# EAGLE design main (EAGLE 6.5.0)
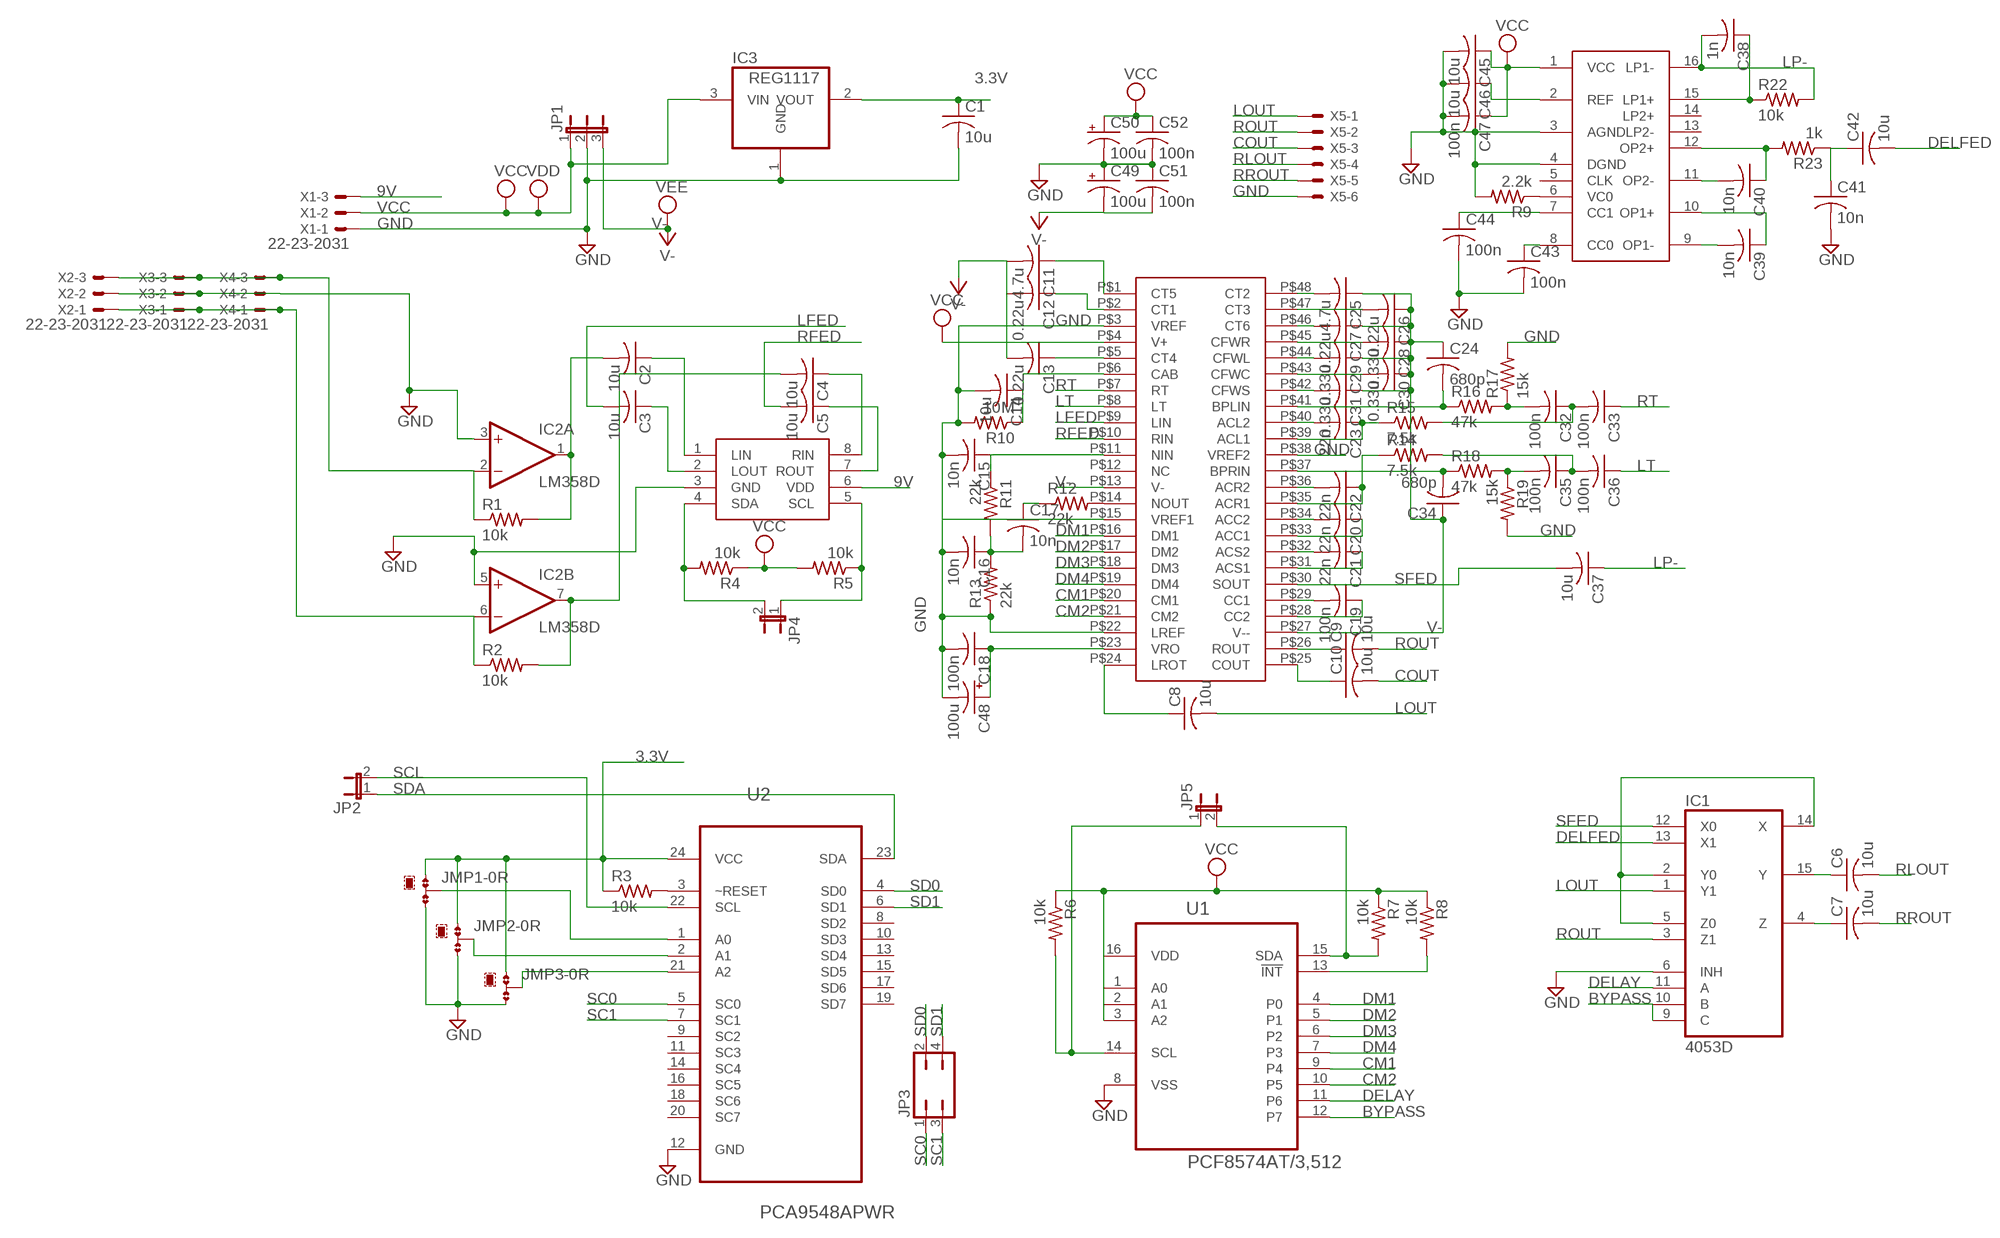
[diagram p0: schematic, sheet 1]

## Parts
C1  10u  C-USC1206  [C1206]
C2  10u  C-USC1206  [C1206]
C3  10u  C-USC1206  [C1206]
C4  10u  C-USC1206  [C1206]
C5  10u  C-USC1206  [C1206]
C6  10u  C-USC1206  [C1206]
C7  10u  C-USC1206  [C1206]
C8  10u  C-USC1206  [C1206]
C9  10u  C-USC1206  [C1206]
C10  10u  C-USC1206  [C1206]
C11  4.7u  C-USC1206  [C1206]
C12  0.22u  C-USC1206  [C1206]
C13  0.22u  C-USC1206  [C1206]
C14  10u  C-USC1206  [C1206]
C15  10n  C-USC1206  [C1206]
C16  10n  C-USC1206  [C1206]
C17  10n  C-USC1206  [C1206]
C18  100n  C-USC1206  [C1206]
C19  100n  C-USC1206  [C1206]
C20  22n  C-USC1206  [C1206]
C21  22n  C-USC1206  [C1206]
C22  22n  C-USC1206  [C1206]
C23  22n  C-USC1206  [C1206]
C24  680p  C-USC1206  [C1206]
C25  4.7u  C-USC1206  [C1206]
C26  0.22u  C-USC1206  [C1206]
C27  0.22u  C-USC1206  [C1206]
C28  0.33u  C-USC1206  [C1206]
C29  0.33u  C-USC1206  [C1206]
C30  0.33u  C-USC1206  [C1206]
C31  0.33u  C-USC1206  [C1206]
C32  100n  C-USC1206  [C1206]
C33  100n  C-USC1206  [C1206]
C34  680p  C-USC1206  [C1206]
C35  100n  C-USC1206  [C1206]
C36  100n  C-USC1206  [C1206]
C37  10u  C-USC1206  [C1206]
C38  1n  C-USC1206  [C1206]
C39  10n  C-USC1206  [C1206]
C40  10n  C-USC1206  [C1206]
C41  10n  C-USC1206  [C1206]
C42  10u  C-USC1206  [C1206]
C43  100n  C-USC1206  [C1206]
C44  100n  C-USC1206  [C1206]
C45  10u  C-USC1206  [C1206]
C46  10u  C-USC1206  [C1206]
C47  100n  C-USC1206  [C1206]
C48  100u  CPOL-USE2-5  [E2-5]
C49  100u  CPOL-USE2-5  [E2-5]
C50  100u  CPOL-USE2-5  [E2-5]
C51  100n  C-USC1206  [C1206]
C52  100n  C-USC1206  [C1206]
IC1  4053D  [SO16]
IC2  LM358D  [SO08]
IC3  REG1117  [SOT223]
JMP1  0R-JUMPB  [B0R-JMP]
JMP2  0R-JUMPB  [B0R-JMP]
JMP3  0R-JUMPB  [B0R-JMP]
JP1  JP2W  [JP2W]
JP2  JP1E  [JP1]
JP3  JP2Q  [JP2Q]
JP4  JP1E  [JP1]
JP5  JP1E  [JP1]
R1  10k  R-US_R1206  [R1206]
R2  10k  R-US_R1206  [R1206]
R3  10k  R-US_R1206  [R1206]
R4  10k  R-US_R1206  [R1206]
R5  10k  R-US_R1206  [R1206]
R6  10k  R-US_R1206  [R1206]
R7  10k  R-US_R1206  [R1206]
R8  10k  R-US_R1206  [R1206]
R9  2.2k  R-US_R1206  [R1206]
R10  10M  R-US_R1206  [R1206]
R11  22k  R-US_R1206  [R1206]
R12  22k  R-US_R1206  [R1206]
R13  22k  R-US_R1206  [R1206]
R14  7.5k  R-US_R1206  [R1206]
R15  7.5k  R-US_R1206  [R1206]
R16  47k  R-US_R1206  [R1206]
R17  15k  R-US_R1206  [R1206]
R18  47k  R-US_R1206  [R1206]
R19  15k  R-US_R1206  [R1206]
R22  10k  R-US_R1206  [R1206]
R23  1k  R-US_R1206  [R1206]
U1  PCF8574AT/3,512  [SOIC127P1032X265-16N]
U2  PCA9548APWR  [SOP65P640X120-24N]
U$1  SSM2126  [DIP48]
U$2  PT2257  [SO08]
U$3  PT2399  [DIL16]
X1  22-23-2031  [22-23-2031]
X2  22-23-2031  [22-23-2031]
X3  22-23-2031  [22-23-2031]
X4  22-23-2031  [22-23-2031]
X5  22-23-2061  [22-23-2061]

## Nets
3.3V: C1.1 IC3.2(VOUT) JMP1.1 JMP2.1 JMP3.1 R3.1 U2.24(VCC)
9V: U$2.6(VDD) X1.3
BYPASS: IC1.9(C) IC1.10(B) U1.12(P7)
CM1: U1.9(P4) U$1.P$20(CM1)
CM2: U1.10(P5) U$1.P$21(CM2)
COUT: C10.2 X5.3
DELAY: IC1.11(A) U1.11(P6)
DELFED: C42.2 IC1.13(X1)
DM1: U1.4(P0) U$1.P$16(DM1)
DM2: U1.5(P1) U$1.P$17(DM2)
DM3: U1.6(P2) U$1.P$18(DM3)
DM4: U1.7(P3) U$1.P$19(DM4)
GND: C1.2 C14.2 C15.2 C16.2 C18.2 C41.2 C43.2 C44.2 C45.2 C46.2 C47.2 C48.- C49.+ C50.- C51.1 C52.2 IC1.6(INH) IC2.3(A:+IN) IC2.5(B:+IN) IC3.1(GND) JMP1.3 JMP2.3 JMP3.3 JP1.2 R9.2 R10.2 R13.1 R17.2 R19.2 U1.8(VSS) U2.12(GND) U$1.P$3(VREF) U$1.P$15(VREF1) U$1.P$22(LREF) U$1.P$38(VREF2) U$2.3(GND) U$3.3(AGND) U$3.4(DGND) X1.1 X2.2 X3.2 X4.2 X5.6
LFED: C3.2 U$1.P$9(LIN)
LOUT: C8.2 IC1.1(Y1) X5.1
LP-: C37.1 C38.2 R22.2 U$3.16(LP1-)
LT: C36.1 U$1.P$8(LT)
N$1: R3.2 U2.3(~RESET)
N$2: C2.2 IC2.1(A:OUT) R1.2
N$3: IC2.2(A:-IN) R1.1 X2.3 X3.3 X4.3
N$4: IC2.6(B:-IN) R2.1 X2.1 X3.1 X4.1
N$5: C4.2 IC2.7(B:OUT) R2.2
N$6: C11.1 U$1.P$1(CT5)
N$7: R9.1 U$3.6(VC0)
N$8: C2.1 U$2.1(LIN)
N$9: C4.1 U$2.8(RIN)
N$10: C3.1 U$2.2(LOUT)
N$11: C5.1 U$2.7(ROUT)
N$12: JMP2.2 U2.2(A1)
N$13: JMP3.2 U2.21(A2)
N$14: JMP1.2 U2.1(A0)
N$15: IC1.2(Y0) IC1.5(Z0) IC1.14(X)
N$16: C6.1 IC1.15(Y)
N$17: C7.1 IC1.4(Z)
N$18: R8.2 U1.13(!INT)
N$19: C8.1 U$1.P$24(LROT)
N$20: C12.1 U$1.P$2(CT1)
N$21: C9.1 U$1.P$26(ROUT)
N$22: C10.1 U$1.P$25(COUT)
N$23: C13.1 U$1.P$5(CT4)
N$24: C14.1 R10.1 U$1.P$6(CAB)
N$25: R12.2 U$1.P$14(NOUT)
N$26: C15.1 R11.1 U$1.P$11(NIN)
N$27: C16.1 C17.2 R11.2 R13.2
N$28: C17.1 R12.1
N$29: C19.2 U$1.P$29(CC1)
N$30: C18.1 C48.+ U$1.P$23(VRO)
N$31: C19.1 U$1.P$28(CC2)
N$32: C21.1 U$1.P$31(ACS1)
N$33: C21.2 U$1.P$32(ACS2)
N$34: C20.1 U$1.P$33(ACC1)
N$35: C20.2 U$1.P$34(ACC2)
N$36: C22.1 R14.1 U$1.P$35(ACR1)
N$37: C22.2 U$1.P$36(ACR2)
N$38: C23.2 U$1.P$40(ACL2)
N$39: C23.1 R15.1 U$1.P$39(ACL1)
N$40: C24.2 R16.1 U$1.P$41(BPLIN)
N$41: C27.2 U$1.P$46(CT6)
N$42: C31.2 U$1.P$42(CFWS)
N$43: C30.2 U$1.P$43(CFWC)
N$44: C29.2 U$1.P$44(CFWL)
N$45: C28.2 U$1.P$45(CFWR)
N$46: C26.2 U$1.P$47(CT3)
N$47: C25.2 U$1.P$48(CT2)
N$49: C32.2 R16.2 R17.1
N$50: C32.1 C33.2 R15.2
N$51: C34.2 R18.1 U$1.P$37(BPRIN)
N$52: C39.2 U$3.9(OP1-)
N$53: C35.2 R18.2 R19.1
N$54: C35.1 C36.2 R14.2
N$55: C38.1 R22.1 U$3.15(LP1+)
N$56: C40.2 U$3.11(OP2-)
N$57: C39.1 U$3.10(OP1+)
N$58: C40.1 R23.2 U$3.12(OP2+)
N$59: C41.1 C42.1 R23.1
N$60: C44.1 U$3.7(CC1)
N$61: C43.1 U$3.8(CC0)
N$62: JP4.2 R4.2 U$2.4(SDA)
N$63: C46.1 U$3.2(REF)
N$64: JP4.1 R5.1 U$2.5(SCL)
N$65: JP5.2 R7.2 U1.15(SDA)
N$67: JP5.1 R6.2 U1.14(SCL)
RFED: C5.2 U$1.P$10(RIN)
RLOUT: C6.2 X5.4
ROUT: C9.2 IC1.3(Z1) X5.2
RROUT: C7.2 X5.5
RT: C33.1 U$1.P$7(RT)
SC0: JP3.1 U2.5(SC0)
SC1: JP3.3 U2.7(SC1)
SCL: JP2.2 U2.22(SCL)
SD0: JP3.2 U2.4(SD0)
SD1: JP3.4 U2.6(SD1)
SDA: JP2.1 U2.23(SDA)
SFED: C37.2 IC1.12(X0) U$1.P$30(SOUT)
V-: C11.2 C12.2 C13.2 C24.1 C25.1 C26.1 C27.1 C28.1 C29.1 C30.1 C31.1 C34.1 C49.- C51.2 JP1.3 U$1.P$13(V-) U$1.P$27(V--) ; supply symbol labelled VEE
VCC: C45.1 C47.1 C50.+ C52.1 IC3.3(VIN) JP1.1 R4.1 R5.2 R6.1 R7.1 R8.1 U1.1(A0) U1.2(A1) U1.3(A2) U1.16(VDD) U$1.P$4(V+) U$3.1(VCC) X1.2 ; supply symbol labelled VDD
Unconnected: U2.8(SD2) U2.9(SC2) U2.10(SD3) U2.11(SC3) U2.13(SD4) U2.14(SC4) U2.15(SD5) U2.16(SC5) U2.17(SD6) U2.18(SC6) U2.19(SD7) U2.20(SC7) U$1.P$12(NC) U$3.5(CLK) U$3.13(LP2-) U$3.14(LP2+)

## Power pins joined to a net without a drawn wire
GND: IC1.8(GND)
V+: IC2.8(P:V+)
V-: IC1.7(VEE) IC2.4(P:V-)
VCC: IC1.16(VCC)

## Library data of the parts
C1-C47 C51 C52 = adafruit:C-US: CAPACITOR, American symbol
C48-C50 = adafruit:CPOL-US: POLARIZED CAPACITOR, American symbol
IC1 = 40xx:4053: Triple 2-channel ANALOG MULTIPLEXER
IC2 = linear:LM358: OP AMP also LM158; LM258; LM2904 Source: http://cache.national.com/ds/LM/LM158.pdf
IC3 = burr-brown:REG1117: 800mA and 1A Low Dropout (LDO) Positive Regulator 1.8V, 2.5V, 2.85V, 3.3V, 5V, and Adj; MPN: REG1117; OC_FARNELL: 1097566; OC_NEWARK: 14P6981
JMP1-JMP3 = jump-0r-smd:0R-JUMP: SMD 0R 0805 Jumper
JP1 = jumper:JP2W: JUMPER
JP2 JP4 JP5 = jumper:JP1E: JUMPER
JP3 = jumper:JP2Q: JUMPER
R1-R19 R22 R23 = adafruit:R-US_: RESISTOR, American symbol
U1 = PCF8574A:PCF8574AT/3,512: IC, I/O EXPANDER, 8BIT, 16SOIC; MPN: PCF8574AT/3,512; OC_FARNELL: 2101302; OC_NEWARK: 70R6866; PACKAGE: SOIC-16; SUPPLIER: NXP
U2 = PCA9548A:PCA9548APWR: 8-CHANNEL I2C SWITCH WITH RESET; MPN: PCA9548APWR False; OC_FARNELL: 1607855; OC_NEWARK: 22M1602; PACKAGE: TSSOP-24; SUPPLIER: Texas Instruments
U$1 = adafruit:SSM2126
U$2 = adafruit:PT2257
U$3 = adafruit:PT2399
X1-X4 = con-molex:22-23-2031: .100" (2.54mm) Center Header - 3 Pin; MF: MOLEX; MPN: 22-23-2031; OC_FARNELL: 1462950; OC_NEWARK: 30C0862
X5 = con-molex:22-23-2061: .100" (2.54mm) Center Header - 6 Pin; MF: MOLEX; MPN: 22-23-2061; OC_FARNELL: 1462922; OC_NEWARK: 27C1933

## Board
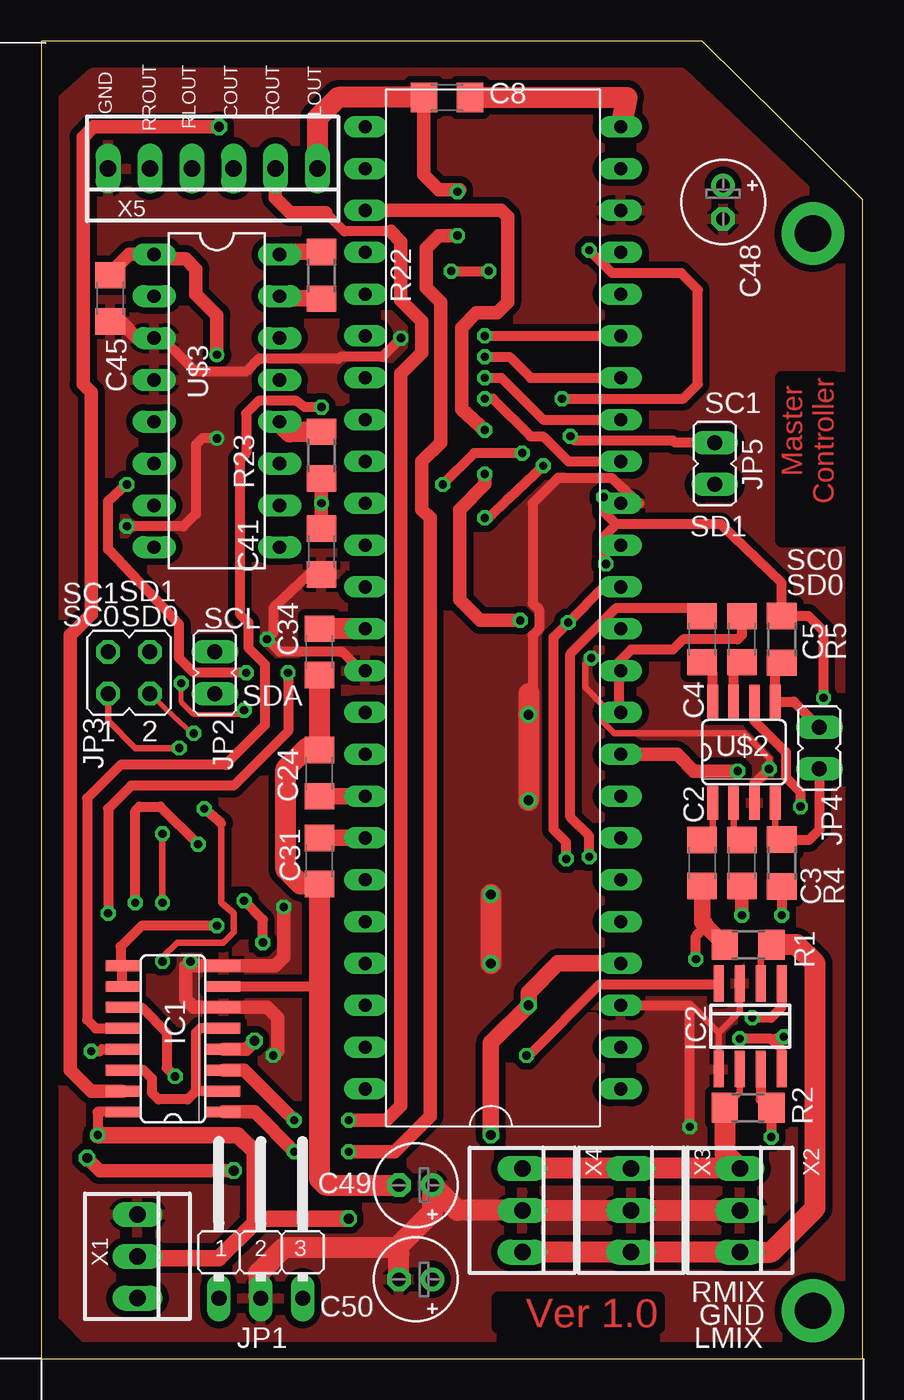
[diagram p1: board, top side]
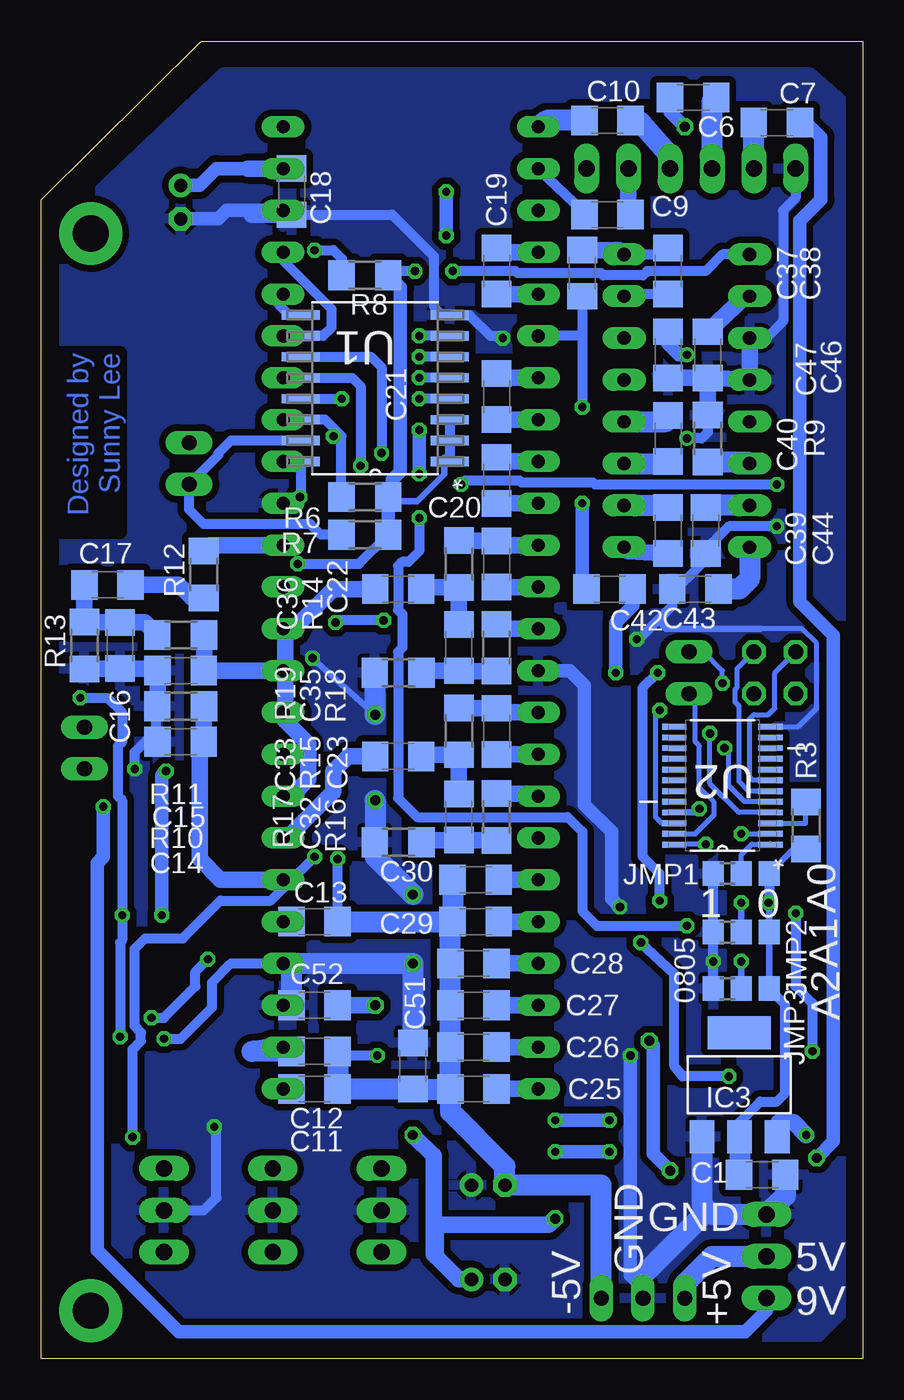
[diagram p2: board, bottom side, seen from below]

Size 49.87 x 80 mm. Coordinates in mm from the lower left corner, seen from the top.
Outline: 0,0 49.87,0 49.87,70.36 40.14,80 0,80 0,0
Copper layers (1*16): Top 0.035mm / dielectric 1.5mm / Bottom 0.035mm
Design rules "default *": minimum track width 10mil, minimum drill 16mil, track to track 6mil, track to pad 6mil, pad to pad 6mil, via to via 6mil, smd to smd 4mil, copper to edge 40mil, drill to drill 8mil, minimum pad ring 10mil, minimum via ring 8mil, stop-mask expansion 4mil, vias tented up to drill 0mil, thermal gap 10mil

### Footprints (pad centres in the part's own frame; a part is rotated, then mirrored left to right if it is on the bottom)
C1206 = smd 1.6 x 1.8: 1 -1.4,0; 2 1.4,0
E2-5 = drill 0.813 pad 1.422: + -1.016,0 | drill 0.813 pad 1.422 octagon: - 1.016,0
SO16 = smd 0.66 x 2.032: 1 -4.445,-3.073; 2 -3.175,-3.073; 3 -1.905,-3.073; 4 -0.635,-3.073; 5 0.635,-3.073; 6 1.905,-3.073; 7 3.175,-3.073; 8 4.445,-3.073; 9 4.445,3.073; 10 3.175,3.073; 11 1.905,3.073; 12 0.635,3.073; 13 -0.635,3.073; 14 -1.905,3.073; 15 -3.175,3.073; 16 -4.445,3.073
SO08 = smd 0.6 x 2.2: 1 -1.905,-2.6; 2 -0.635,-2.6; 3 0.635,-2.6; 4 1.905,-2.6; 5 1.905,2.6; 6 0.635,2.6; 7 -0.635,2.6; 8 -1.905,2.6
SOT223 = smd 1.499 x 2.007: 1 -2.261,-3.15; 2 0.025,-3.15; 3 2.311,-3.15 | smd 3.81 x 2.007: 4 0,3.15
B0R-JMP = smd 1.5 x 1.3: 1 0,1.7; 2 0,0; 3 0,-1.7
JP2W = drill 0.914 long: 1 -2.54,-1.27; 2 0,-1.27; 3 2.54,-1.27
JP1 = drill 0.914 long: 1 0,-1.27; 2 0,1.27
JP2Q = drill 0.914 octagon: 1 -1.27,-1.27; 2 1.27,-1.27; 3 -1.27,1.27; 4 1.27,1.27
R1206 = smd 1.6 x 1.803: 1 -1.422,0; 2 1.422,0
SOIC127P1032X265-16N = smd 2.286 x 0.559: 1 -4.521,4.445; 2 -4.521,3.175; 3 -4.521,1.905; 4 -4.521,0.635; 5 -4.521,-0.635; 6 -4.521,-1.905; 7 -4.521,-3.175; 8 -4.521,-4.445; 9 4.521,-4.445; 10 4.521,-3.175; 11 4.521,-1.905; 12 4.521,-0.635; 13 4.521,0.635; 14 4.521,1.905; 15 4.521,3.175; 16 4.521,4.445
SOP65P640X120-24N = smd 1.473 x 0.356: 1 -2.921,3.581; 2 -2.921,2.921; 3 -2.921,2.286; 4 -2.921,1.626; 5 -2.921,0.965; 6 -2.921,0.33; 7 -2.921,-0.33; 8 -2.921,-0.965; 9 -2.921,-1.626; 10 -2.921,-2.286; 11 -2.921,-2.921; 12 -2.921,-3.581; 13 2.921,-3.581; 14 2.921,-2.921; 15 2.921,-2.286; 16 2.921,-1.626; 17 2.921,-0.965; 18 2.921,-0.33; 19 2.921,0.33; 20 2.921,0.965; 21 2.921,1.626; 22 2.921,2.286; 23 2.921,2.921; 24 2.921,3.581
DIP48 = drill 0.8 long: P$1 -29.21,-8.89; P$2 -26.67,-8.89; P$3 -24.13,-8.89; P$4 -21.59,-8.89; P$5 -19.05,-8.89; P$6 -16.51,-8.89; P$7 -13.97,-8.89; P$8 -11.43,-8.89; P$9 -8.89,-8.89; P$10 -6.35,-8.89; P$11 -3.81,-8.89; P$12 -1.27,-8.89; P$13 1.27,-8.89; P$14 3.81,-8.89; P$15 6.35,-8.89; P$16 8.89,-8.89; P$17 11.43,-8.89; P$18 13.97,-8.89; P$19 16.51,-8.89; P$20 19.05,-8.89; P$21 21.59,-8.89; P$22 24.13,-8.89; P$23 26.67,-8.89; P$24 29.21,-8.89; P$25 29.21,6.604; P$26 26.67,6.604; P$27 24.13,6.604; P$28 21.59,6.604; P$29 19.05,6.604; P$30 16.51,6.604; P$31 13.97,6.604; P$32 11.43,6.604; P$33 8.89,6.604; P$34 6.35,6.604; P$35 3.81,6.604; P$36 1.27,6.604; P$37 -1.27,6.604; P$38 -3.81,6.604; P$39 -6.35,6.604; P$40 -8.89,6.604; P$41 -11.43,6.604; P$42 -13.97,6.604; P$43 -16.51,6.604; P$44 -19.05,6.604; P$45 -21.59,6.604; P$46 -24.13,6.604; P$47 -26.67,6.604; P$48 -29.21,6.604
SO08' = smd 0.66 x 2.032: 1 -1.905,-3.073; 2 -0.635,-3.073; 3 0.635,-3.073; 4 1.905,-3.073; 5 1.905,3.073; 6 0.635,3.073; 7 -0.635,3.073; 8 -1.905,3.073
DIL16 = drill 0.813 long: 1 -8.89,-3.81; 2 -6.35,-3.81; 3 -3.81,-3.81; 4 -1.27,-3.81; 5 1.27,-3.81; 6 3.81,-3.81; 7 6.35,-3.81; 8 8.89,-3.81; 9 8.89,3.81; 10 6.35,3.81; 11 3.81,3.81; 12 1.27,3.81; 13 -1.27,3.81; 14 -3.81,3.81; 15 -6.35,3.81; 16 -8.89,3.81
22-23-2031 = drill 1 long: 1 -2.54,0; 2 0,0; 3 2.54,0
22-23-2061 = drill 1 long: 1 -6.35,0; 2 -3.81,0; 3 -1.27,0; 4 1.27,0; 5 3.81,0; 6 6.35,0

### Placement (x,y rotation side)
C1  6.1,11.18 0 bottom
C2  40.13,30.1 270 top
C3  42.55,30.1 270 top
C4  40.13,43.69 90 top
C5  42.55,43.69 90 top
C6  10.29,76.58 0 bottom
C7  5.21,75.06 180 bottom
C8  24.64,76.58 180 top
C9  15.49,69.47 0 bottom
C10  15.49,75.18 0 bottom
C11  33.27,16.38 0 bottom
C12  33.27,18.67 0 bottom
C13  33.27,26.54 0 bottom
C14  41.4,37.47 180 bottom
C15  41.4,41.78 180 bottom
C16  45.09,43.31 270 bottom
C17  45.85,46.99 180 bottom
C18  34.67,70.87 270 bottom
C19  22.23,66.04 270 bottom
C20  22.23,53.34 270 bottom
C21  22.23,58.42 270 bottom
C22  22.23,48.26 270 bottom
C23  22.23,38.1 270 bottom
C24  16.89,35.56 270 top
C25  23.62,16.38 0 bottom
C26  23.62,18.92 0 bottom
C27  23.62,21.46 0 bottom
C28  23.62,24 0 bottom
C29  23.5,26.54 0 bottom
C30  23.5,29.08 0 bottom
C31  16.89,30.23 90 top
C32  24.51,32.89 270 bottom
C33  28.19,36.58 0 bottom
C34  16.89,42.93 90 top
C35  24.51,43.18 270 bottom
C36  28.19,46.74 0 bottom
C37  17.02,65.91 270 bottom
C38  11.81,66.04 90 bottom
C39  11.81,50.29 270 bottom
C40  11.81,55.88 270 bottom
C41  17.02,49.02 270 top
C42  15.37,46.74 0 bottom
C43  10.16,46.74 180 bottom
C44  9.53,50.29 270 bottom
C45  4.19,64.39 270 top
C46  9.4,60.96 270 bottom
C47  11.81,60.96 270 bottom
C48  41.4,70.23 270 top
C49  22.73,10.54 180 top
C50  22.73,4.83 180 top
C51  27.3,17.78 270 bottom
C52  33.27,21.46 180 bottom
IC1  8,19.43 90 top
IC2  43.05,20.19 180 top
IC3  7.49,16.64 0 bottom
JMP1  7.37,29.46 270 bottom
JMP2  7.37,25.91 270 bottom
JMP3  7.37,22.48 270 bottom
JP1  13.34,4.95 0 top
JP2  10.54,41.66 0 top
JP3  5.33,41.66 0 top
JP4  47.24,37.08 180 top
JP5  40.89,54.36 180 top
R1  42.93,25.15 180 top
R2  42.93,15.24 0 top
R3  3.43,32.38 90 bottom
R4  44.96,30.1 90 top
R5  44.96,43.69 90 top
R6  30.23,52.32 180 bottom
R7  30.23,50.04 180 bottom
R8  30.23,65.79 180 bottom
R9  9.4,55.88 90 bottom
R10  41.4,39.62 180 bottom
R11  41.4,43.94 180 bottom
R12  40.01,47.62 90 bottom
R13  47.24,43.31 90 bottom
R14  24.51,48.26 270 bottom
R15  24.51,38.1 270 bottom
R16  22.23,32.89 270 bottom
R17  28.19,31.37 180 bottom
R18  22.23,43.18 270 bottom
R19  28.19,41.66 180 bottom
R22  17.02,65.79 90 top
R23  17.02,54.86 90 top
U1  29.59,58.93 180 bottom
U2  8.51,34.8 180 bottom
U$1  26.29,45.59 90 top
U$2  PT2257  [SO08']  42.67,36.83 0 top
U$3  10.67,58.17 270 top
X1  5.84,6.22 270 top
X2  42.42,9.02 270 top
X3  35.81,9.02 270 top
X4  29.21,9.02 270 top
X5  10.41,72.26 180 top

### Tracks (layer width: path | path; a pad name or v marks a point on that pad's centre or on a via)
3.3V  (via drill 0.5)
  Top 0.61: v5.71,27.69 5.71,33.27 5.97,33.53 7.24,33.53 v9.53,31.24
  Bottom 0.305: v9.53,31.24 11.4,31.24 U2.24
  Bottom 0.406: JMP3.1 JMP2.1 JMP1.1 4.17,30.96 R3.1
  Bottom 0.61: IC3.2 7.47,14.38 6.22,15.62 5.21,15.62 4.7,16.13 4.7,21.51 JMP3.1 | JMP1.1 5.67,27.73 v5.71,27.69
  Bottom 1.27: IC3.2 7.47,11.2 C1.1
9V  (via drill 0.5)
  Top 0.61: U$2.6 43.31,38.73 45.21,36.83 45.21,35.31 46.1,34.42 v46.1,33.53
  Bottom 0.61: 7.24,1.52 7.11,1.65
  Bottom 0.813: X1.3 5.84,2.92 7.11,1.65 41.53,1.65 46.48,6.6 46.48,30.1 46.1,30.48 v46.1,33.53
BYPASS  (via drill 0.5)
  Top 0.61: IC1.10 IC1.9 4.83,23.98 4.83,25.02 6.1,26.29 v10.67,26.29 | v30.48,54.23 28.32,52.2 27.18,51.05 v26.92,51.05
  Bottom 0.61: U1.12 30.99,59.56 30.48,59.05 v30.48,54.23 | v26.92,51.05 26.92,49.02 27.56,48.39 27.94,48.39 28.19,48.13 28.19,45.47 27.94,45.21 27.94,43.18 28.19,42.93 28.19,34.04 27.05,32.89 17.91,32.89 17.02,32 17.02,27.18 16.13,26.29 v10.67,26.29
CM1
  Bottom 0.61: U1.9 34.8,63.37 36.07,64.64 U$1.P$20
CM2
  Bottom 0.61: U$1.P$21 35.69,67.18 32.26,63.75 32.26,62.61 32.77,62.1 U1.10
COUT
  Bottom 1.27: C10.2 13.46,75.06 11.68,73.03 X5.3
DELAY  (via drill 0.5)
  Top 0.61: v29.21,54.99 26.29,54.99 v24.38,53.09 | IC1.11 6.1,21.34 7.62,19.81 7.62,17.65 v8.13,17.14 | v13.46,25.27 13.46,26.67 v12.32,27.81 | v12.45,41.66 9.27,41.66 8.38,42.55 8.38,44.58 4.06,49.15 4.06,52.07 v5.21,53.09
  Bottom 0.61: U1.11 29.84,60.83 29.21,60.2 v29.21,54.99 | v24.38,53.09 24.13,53.34 20.83,53.34 20.7,53.21 16.38,53.21 16.26,53.09 v5.21,53.09 | v8.13,17.14 10.92,17.14 11.43,17.78 11.43,23.37 v13.46,25.27 | v12.32,27.81 12.32,29.46 13.34,30.48 13.34,40.77 v12.45,41.66
DELFED  (via drill 0.5)
  Top 0.61: v14.99,41.66 14.99,38.1 11.68,34.8 5.46,34.8 4.06,33.4 v4.06,27.05 | v3.05,18.67 3.56,18.67 3.68,18.8 IC1.13
  Bottom 0.61: C42.2 13.97,45.84 | v4.06,27.05 4.06,22.61 3.05,21.59 v3.05,18.67
  Bottom 0.813: 13.97,45.84 13.97,45.72 14.99,44.7 v14.99,41.66
DM1  (via drill 0.5)
  Top 0.61: v26.92,58.29 27.43,58.29 29.72,56.01 30.48,56.01 32,54.48 U$1.P$16
  Bottom 0.61: U1.4 v26.92,58.29
DM2  (via drill 0.5)
  Top 0.61: v26.92,59.56 27.94,59.56 30.48,57.02 U$1.P$17
  Bottom 0.61: U1.5 v26.92,59.56
DM3  (via drill 0.5)
  Top 0.61: v26.92,60.83 28.45,60.83 29.72,59.56 U$1.P$18
  Bottom 0.61: U1.6 v26.92,60.83
DM4  (via drill 0.5)
  Top 0.61: v26.92,62.1 U$1.P$19
  Bottom 0.61: U1.7 v26.92,62.1
GND  (via drill 0.5, 0.6)
  Top 0.406: U$2.3 43.31,33.66 43.43,33.53 43.43,35.05 v44.2,35.81 44.2,36.45 42.67,37.97 34.8,37.97 34.16,38.61 34.16,39.62 33.02,40.77 33.02,42.16 v33.4,42.55 | IC2.3 42.42,21.08 41.15,19.81 | 41.15,19.81 IC2.5 | 39.37,21.46 39.5,21.46 41.15,19.81
  Top 0.61: U$1.P$3 39.37,21.46 v39.37,14.1 | U$2.3 43.31,34.92 v44.2,35.81 | U$1.P$15 36.32,51.94 34.67,53.47 31.37,53.47 29.84,51.94 29.84,45.85 30.23,45.47 30.23,44.32 29.84,43.94 29.84,40.49 29.62,40.26 | v21.84,61.98 20.7,60.83 18.16,60.83 18.03,60.71 13.21,60.71 12.45,59.94 9.4,59.94 7.37,61.98 | 8.76,23.83 v9.07,24.13 | IC1.8 10.54,23.88 | C41.2 16.25,47.62 14.1,45.59 14.1,44.07 v13.72,43.69 14.48,42.93 18.29,42.93 19.43,41.78 U$1.P$38 | v10.67,55.88 9.78,55.88 9.4,55.5 9.4,51.31 8.64,50.55 v5.21,50.55
  Top 0.813: C45.2 4.83,62.99 5.84,61.98 U$3.3 | 8.76,23.83 8.76,21.84 9.27,21.34 IC1.6 13.72,21.34 14.35,20.7 14.35,18.67 v14.1,18.41 | v9.07,24.13 9.32,23.88 10.54,23.88 14.22,23.88 14.73,24.38 v14.73,27.43
  Top 1.016: 7.37,61.98 U$3.3
  Top 1.27: X2.2 X3.2 X4.2 25.27,9.02 C49.+ 23.75,8.89 21.72,6.86 C50.- 21.72,6.35 21.34,6.73 14.73,6.73 13.21,5.21 13.21,3.81 JP1.2 | v27.3,28.19 v27.3,24 | v29.59,33.91 v29.59,39.12 29.62,39.14 29.62,40.26 29.62,40.39
  Bottom 0.305: U2.12 3.91,38.38 2.79,39.5 2.79,43.43 3.68,44.32 6.22,44.32
  Bottom 0.406: v33.4,42.55 v29.59,39.12 | 6.22,44.32 11.94,44.32 12.45,44.83
  Bottom 0.61: v44.2,35.81 44.2,36.83 43.43,37.59 42.93,37.59 C14.2 42.93,37.59 42.93,41.91 | X2.2 40.01,9.02 39.24,9.78 39.24,13.97 v39.37,14.1 | JMP3.3 v9.07,24.13 JMP2.3 JMP1.3 | C18.2 28.57,69.47 26.04,66.93 26.04,63.88 25.6,63.45 25.15,63.45 U1.8 23.88,63.37 22.61,62.1 22.1,62.1 v21.84,61.98 | v13.72,43.69 13.59,43.69 12.45,44.83 11.56,45.72 C43.2 11.3,46.74 9.65,48.39 9.65,48.89 C44.2 9.4,49.02 9.4,49.28 8.13,50.55 v5.21,50.55 | R9.2 9.4,56.26 9.78,55.88 v10.67,55.88 | X5.6 4.06,70.48 4.83,69.72 4.83,62.99 5.84,61.98 U$3.3
  Bottom 0.813: U$1.P$22 38.61,69.72 39.12,69.22 C48.- | v14.1,18.41 14.1,5.08 13.34,4.32 | U$1.P$38 17.78,41.78 16.89,40.89 16.89,33.66 15.24,32 15.24,27.94 v14.73,27.43
  Bottom 1.016: R13.1 45.11,41.88 C16.2 42.93,41.91 C15.2 42.8,39.65 R10.2 | C18.2 37.08,69.47 U$1.P$22 | C47.2 C46.2 | C46.2 R9.2 | C46.2 U$3.4 U$3.3
  Bottom 1.27: C1.2 4.7,9.91 X1.1 9.14,8.76 9.4,9.02 | IC3.1 9.75,9.37 9.4,9.02 | JP1.2 13.34,4.32 13.34,5.08 9.4,9.02 | U$1.P$3 C52.2 34.67,24 v27.3,24 C51.1 | v27.3,28.19 29.62,30.5 R17.2 29.59,31.39 v29.59,33.91 | R19.2 29.62,39.14 v29.59,39.12
  pour Top (isolate 0.406): 48.51,0.76 3.17,0.76 1.27,2.67 1.27,76.45 3.17,78.11 38.86,78.11 48.51,68.96
  pour Bottom (isolate 0.406): 48.51,0.76 3.17,0.76 1.27,2.67 1.27,76.45 3.17,78.11 38.86,78.11 48.51,68.96
LFED  (via drill 0.5)
  Top 0.813: C3.2 v42.55,26.92 | v42.29,35.69 39.62,35.69 38.61,36.7 U$1.P$9
  Bottom 0.813: v42.55,26.92 42.55,35.43 v42.29,35.69
LOUT  (via drill 0.5)
  Top 0.61: v25.27,70.87 25.4,70.99
  Top 0.813: IC1.1 12.95,14.99 v15.37,12.57 | v18.67,12.57 21.46,12.57 23.62,14.73 23.62,51.05 23.11,51.56 23.11,54.48 24.26,55.63 24.26,64.14 23.37,65.02 23.37,67.44 24.13,68.2 v25.27,68.2 | 25.4,70.99 24.13,70.99 23.24,71.88 C8.2
  Top 1.27: C8.2 18.03,76.58 16.76,75.31 X5.1
  Bottom 0.813: v15.37,12.57 v18.67,12.57 | v25.27,68.2 v25.27,70.87
LP-
  Top 1.016: R22.2 14.5,67.21 U$3.16
  Bottom 0.61: U$3.16 12.2,67.06 C38.2
  Bottom 1.016: C37.1 14.73,67.31 U$3.16
LT
  Bottom 1.016: C36.1 32.13,46.74 35.05,43.81 35.05,38.73 33.66,37.34 33.66,35.18 34.67,34.16 U$1.P$8
N$1
  Bottom 0.305: U2.3 3.45,32.51 R3.2
N$2  (via drill 0.5)
  Top 0.61: IC2.1 44.96,21.34 44.32,20.7 v43.18,20.7 | 40.44,26.21 40.44,26.62 40.13,26.92 | v39.75,24.26 39.75,25.65 40.37,26.28
  Top 1.016: C2.2 40.13,26.92 40.13,26.52 40.37,26.28 40.44,26.21 R1.2
  Bottom 0.61: v43.18,20.7 42.42,20.7 40.51,22.61 40.51,23.5 v39.75,24.26
N$3
  Top 0.406: IC2.2 43.69,24.49 R1.1
  Top 1.27: X4.3 X3.3 X2.3 44.32,6.48 46.99,9.14 46.99,24 45.85,25.15 R1.1
N$4
  Top 0.406: IC2.6 42.42,16.15 R2.1
  Top 1.27: X4.1 X3.1 X2.1 41.5,12.47 R2.1
N$5  (via drill 0.5)
  Top 0.406: IC2.7 43.69,15.9 R2.2
  Top 0.61: IC2.7 43.69,15.75 44.32,15.11 v44.32,13.46 | v33.27,30.48 33.27,31.75 32.13,32.89 32.13,42.8 34.92,45.59 39.63,45.59 C4.2
  Bottom 0.61: v44.32,13.46 44.32,18.8 43.81,19.3 43.81,19.81 44.2,20.19 44.2,24.89 43.56,25.53 41.27,25.53 38.99,27.81 35.94,27.81 v33.27,30.48
N$6
  Bottom 1.27: C11.1 U$1.P$1
N$7
  Bottom 1.27: R9.1 7.01,54.46 U$3.6
N$8
  Top 0.406: U$2.1 40.77,31.88 C2.1
N$9
  Top 0.61: U$2.8 40.77,41.65 C4.1
N$10
  Top 0.406: U$2.2 42.04,32.01 C3.1
N$11
  Top 0.61: U$2.7 42.04,41.78 C5.1
N$12  (via drill 0.5)
  Top 0.406: v7.37,27.69 v7.37,31.88
  Bottom 0.305: v7.37,31.88 U2.2
  Bottom 0.406: JMP2.2 v7.37,27.69
N$13  (via drill 0.5)
  Top 0.406: 10.92,32.51 10.92,27.69 11.68,27.05 11.68,25.91 11.05,25.27 8.26,25.27 7.37,24.38 v7.37,24.13
  Top 0.61: 10.92,32.51 v9.91,33.4
  Bottom 0.406: U2.21 10.19,33.17 v9.91,33.4 | v7.37,24.13 JMP3.2
N$14
  Bottom 0.305: JMP1.2 7.37,30.61 6.73,31.24 5.61,31.24
  Bottom 0.406: 5.61,31.24 U2.1
N$15
  Top 0.61: IC1.2 9.4,16.26 | IC1.5 9.65,20.07 9.4,19.81 9.4,16.26 | 9.4,16.26 8.89,15.75 7.11,15.75 6.73,16.13 6.73,17.02 6.22,17.53 IC1.14
N$16  (via drill 0.6)
  Top 0.813: v10.79,74.8 3.17,74.8 2.54,74.17 2.54,59.18 3.05,58.67 3.05,45.21 1.78,43.94 1.78,17.53 3.05,16.26 IC1.15
  Bottom 0.61: C6.1 11.69,75.69
  Bottom 0.813: 11.69,75.69 v10.79,74.8
N$17  (via drill 0.6)
  Top 0.813: IC1.4 12.45,18.8 v12.95,19.3 | v11.68,11.43 3.56,11.43 v2.79,12.19
  Bottom 0.61: 3.17,74.8 3.55,74.8 C7.1
  Bottom 0.813: v12.95,19.3 12.7,19.05 12.7,12.45 v11.68,11.43 | v2.79,12.19 1.78,13.21 1.78,43.94 3.81,45.97 3.81,69.09 2.54,70.36 2.54,74.17 3.17,74.8
N$18  (via drill 0.5)
  Top 0.61: v31.62,58.29 38.99,58.29 39.88,59.18 39.88,64.9 38.86,65.91 34.67,65.91 v33.27,67.31
  Bottom 0.61: U1.13 v31.62,58.29 | v33.27,67.31 32.13,67.31 31.62,66.8 31.62,65.81 R8.2
N$19
  Top 1.27: C8.1 35.56,76.58 U$1.P$24
N$20
  Bottom 1.27: C12.1 37.08,18.67 U$1.P$2
N$21
  Bottom 0.61: C9.1 16.89,69.6 U$1.P$26
N$22
  Bottom 1.27: C10.1 19.18,75.18 U$1.P$25
N$23
  Bottom 1.27: C13.1 U$1.P$5
N$24
  Bottom 1.016: R10.1 40,39.6 C14.1 40.26,37.21 40.26,30.35 38.99,29.08 U$1.P$6
N$25
  Bottom 1.016: U$1.P$14 39.65,49.4 R12.2
N$26
  Bottom 1.016: R11.1 39.98,41.8 C15.1 U$1.P$11
N$27
  Bottom 1.016: C17.2 R13.2 45.11,44.73 C16.1 43.59,44.71 R11.2
N$28
  Bottom 1.016: R12.1 40.74,46.2 41.53,46.99 C17.1
N$29
  Bottom 1.016: U$1.P$29 C19.2
N$30
  Bottom 0.813: U$1.P$23 39.24,72.26 40.26,71.25 C48.+
  Bottom 1.016: C18.1 37.34,72.27 U$1.P$23
N$31
  Bottom 1.016: U$1.P$28 21.97,67.18 C19.1
N$32
  Bottom 1.016: U$1.P$31 21.97,59.56 C21.1
N$33
  Bottom 1.016: U$1.P$32 C21.2
N$34
  Bottom 1.016: U$1.P$33 21.97,54.48 C20.1
N$35
  Bottom 1.016: C20.2 19.56,51.94 U$1.P$34
N$36
  Bottom 1.016: U$1.P$35 21.97,49.4 C22.1 24.49,49.66 R14.1
N$37
  Bottom 1.016: C22.2 19.56,46.86 U$1.P$36
N$38
  Bottom 1.016: C23.2 19.56,36.7 U$1.P$40
N$39
  Bottom 1.016: U$1.P$39 21.97,39.24 C23.1 24.49,39.5 R15.1
N$40
  Top 1.016: U$1.P$41 C24.2
  Bottom 1.016: R16.1 19.71,34.31 U$1.P$41
N$41
  Bottom 1.016: U$1.P$46 C27.2
N$42
  Top 1.016: U$1.P$42 C31.2
N$43
  Bottom 1.016: U$1.P$43 C30.2
N$44
  Bottom 1.016: U$1.P$44 C29.2
N$45
  Bottom 1.016: U$1.P$45 C28.2
N$46
  Bottom 1.016: U$1.P$47 C26.2
N$47
  Bottom 1.016: U$1.P$48 C25.2
N$49
  Bottom 1.016: R16.2 24.49,31.47 C32.2 26.65,31.49 R17.1
N$50
  Bottom 1.016: C32.1 R15.2 26.26,36.68 26.29,36.7 26.67,36.7 C33.2
N$51
  Top 1.27: U$1.P$37 C34.2
  Bottom 1.016: U$1.P$37 21.95,44.32 R18.1
N$52
  Bottom 1.016: C39.2 14.22,49.02 U$3.9
N$53
  Bottom 1.016: R18.2 24.49,41.76 C35.2 26.65,41.78 R19.1
N$54
  Bottom 1.016: C35.1 R14.2 26.69,46.84 C36.2
N$55
  Top 1.016: R22.1 17.17,64.49 17.27,64.39 14.61,64.39 U$3.15
  Bottom 0.61: C38.1 14.35,64.64 U$3.15
N$56
  Bottom 1.27: U$3.11 11.94,54.36 C40.2
N$57
  Bottom 1.27: U$3.10 11.81,51.82 C39.1
N$58
  Top 1.27: R23.2 15.11,56.26 14.5,56.87 14.5,56.92 U$3.12
  Bottom 1.27: U$3.12 11.94,56.9 C40.1
N$59  (via drill 0.5)
  Top 0.813: R23.1 v17.02,51.94 C41.1
  Bottom 0.813: v17.02,51.94 17.02,46.99 C42.1
N$60
  Bottom 1.27: U$3.7 9.52,51.82 C44.1
N$61
  Bottom 1.27: U$3.8 6.86,47.37 7.49,46.74 C43.1
N$62
  Top 0.406: U$2.4 44.58,31.65 R4.2
  Top 0.61: JP4.2 47.24,32.13 46.61,31.5 44.98,31.5 R4.2
N$63
  Bottom 1.016: U$3.2 7.12,64.52 C46.1
N$64
  Top 0.61: R5.1 44.58,41.88 U$2.5 45.7,39.9 JP4.1
N$65
  Bottom 0.61: R7.2 32.89,50.04 33.53,50.67 40.01,50.67 40.89,51.56 JP5.2 39.12,54.86 39.12,54.99 38.35,55.75 U1.15
N$66  (via drill 2.2 pad 3.81)
  other vias: 46.86,68.33
N$67  (via drill 0.5)
  Top 0.61: JP5.1 38.48,55.63 38.35,55.75 32.38,55.75 v32.13,56.01
  Bottom 0.61: R6.2 31.65,56.03 31.88,56.26 | 31.88,56.26 32.64,57.02 U1.14 | v32.13,56.01 31.88,56.26
N$68  (via drill 2.2 pad 3.81)
  other vias: 46.86,2.92
RFED
  Top 0.61: C5.2 42.55,43.94 42.29,43.69 38.99,43.69 38.35,43.05 35.81,43.05 35.05,42.29 35.05,39.75 35.56,39.24 U$1.P$10
RLOUT
  Bottom 1.27: X5.4 9.14,76.32 C6.2
ROUT  (via drill 0.5)
  Top 0.61: 21.21,68.45 18.41,68.45 17.27,69.6
  Top 0.813: IC1.3 12.32,17.53 v15.37,14.48 | v18.67,14.48 20.95,14.48 21.84,15.37 21.84,59.82 23.11,61.09 23.11,62.99 21.84,64.26 21.84,67.82 21.21,68.45 | 17.27,69.6 15.11,69.6 14.22,70.48 X5.2
  Bottom 0.813: v15.37,14.48 v18.67,14.48
  Bottom 1.016: X5.2 14.22,69.6 C9.2
RROUT
  Bottom 1.27: X5.5 C7.2
RT
  Bottom 1.016: U$1.P$7 34.92,31.62 32.13,34.42 32.13,35.69 31.24,36.58 C33.1
SC0  (via drill 0.5)
  Top 0.406: v8.38,37.08 5.71,37.08 4.06,38.73 JP3.1
  Bottom 0.305: U2.5 7.16,33.83 8.13,34.8 8.13,37.21
  Bottom 0.406: 8.13,37.21 v8.38,37.08
SC1
  Bottom 0.305: U2.7 6.68,35.13 6.86,35.31 6.86,38.86 6.6,39.12 5.71,39.12 5.33,39.5 5.33,41.66 JP3.3
SCL  (via drill 0.5)
  Top 0.305: v12.32,39.37 12.06,39.12 9.27,39.12 8.51,39.88 v8.51,41.02
  Bottom 0.305: U2.22 12.19,32.51 12.57,32.89 12.57,39.12 v12.32,39.37 | v8.51,41.02 8.51,41.78 9.65,42.93 JP2.2
SD0  (via drill 0.5)
  Top 0.305: v9.27,37.97 9.14,37.97 7.62,39.37 JP3.2
  Bottom 0.305: U2.4 7.52,33.17 9.27,34.92 v9.27,37.97
SD1
  Bottom 0.305: U2.6 6.91,34.47 7.49,35.05 7.49,38.48 7.49,39.62 7.75,39.88 7.75,40.64 7.62,40.77 7.62,41.91 JP3.4
SDA
  Bottom 0.305: U2.23 10.16,31.88 9.02,33.02 9.02,33.78 9.91,34.67 9.91,37.21 10.16,37.47 10.16,40.01 JP2.1
SFED  (via drill 0.5 pad 0.25)
  Top 0.61: v17.02,57.78 16,57.78 15.49,58.17 13.21,58.17 12.45,57.4 12.45,54.99 12.06,54.61 12.06,45.21 12.57,44.7 12.57,43.18 13.59,42.16 13.59,38.48 11.18,36.07 4.83,36.07 2.79,34.04 2.79,20.57 3.3,20.07 IC1.12
  Top 1.016: 19.53,62.13 U$1.P$30
  Bottom 0.61: 17.02,62.1 U$1.P$30 | 17.02,62.1 v17.02,57.78 | C37.2 17.02,62.1
V-  (via drill 0.5)
  Top 0.61: IC1.7 16.76,22.61 16.89,22.73 | v31.88,30.35 31.88,31.37 31.11,32.13 31.11,43.81 v32,44.7 34.16,46.86 U$1.P$13 | v29.46,18.41 29.59,18.41 33.91,22.73 41.09,22.73 IC2.4
  Top 0.813: U$1.P$27 27.94,69.72 28.32,69.34 28.32,64.14 27.69,63.5 26.42,63.5 25.53,62.61 25.53,57.66 v26.92,56.39 | v26.92,53.72 26.92,53.09 25.4,51.56 25.4,46.1 26.67,44.83 v29.08,44.83
  Top 1.27: C34.1 C24.1 16.77,37.08 16.13,37.08 14.86,35.81 14.86,29.72 15.75,28.83 C31.1 16.89,22.73 16.89,10.92 17.27,10.54 C49.-
  Bottom 0.61: C13.2 31.87,29.08 v31.88,30.35 | v29.46,18.41 31.62,18.41 C12.2 | v29.08,44.83 31.88,44.83 v32,44.7
  Bottom 0.813: v26.92,56.39 v26.92,53.72
  Bottom 1.016: C30.1 C29.1
  Bottom 1.27: C25.1 C51.2 C11.2 C12.2 | C25.1 C26.1 C27.1 C28.1 25.02,26.42 C29.1 C13.2 | C30.1 24.89,26.92 25.02,26.8 25.02,26.42 | JP1.3 15.88,10.54 C49.- 21.72,11.68 25.02,14.99 C25.1
VCC  (via drill 0.5, 0.5 pad 0.2, 0.6)
  Top 0.61: 34.92,50.67 41.27,50.67 44.96,47.12 R5.2 46.58,45.11 47.5,44.2 v47.5,40.13 | 34.92,50.67 34.16,49.91 34.16,48.39 v34.29,48.26 | v34.16,52.32 34.16,51.44 34.92,50.67 | v24.89,66.04 v27.18,66.04 | IC1.16 3.43,14.99 v3.43,13.59 | 7.11,66.8 U$3.1 | IC2.8 44.96,18.8 44.39,19.37 | 44.39,19.37 44.32,19.43 v42.42,19.43 | 5.97,6.1 X1.2 | R4.1 v44.96,26.92 | v45.09,19.56 44.39,19.37
  Top 0.813: C45.1 4.19,65.91 5.33,67.06 U$3.1 | v10.67,60.96 10.67,63.37 9.4,64.64 9.4,66.17 8.76,66.8 7.11,66.8
  Top 1.016: v3.43,13.59 11.94,13.59 12.95,12.57 12.95,8.76 | 12.95,8.76 12.95,8.26 10.79,6.1 5.97,6.1 | U$1.P$4 31.37,24 29.59,22.23 v29.59,21.46 27.3,19.18 v27.3,13.59 | v18.67,8.51 13.21,8.51 12.95,8.76
  Bottom 0.406: 25.4,54.61 25.4,53.72 27.05,52.07 28.55,52.07 R6.1 | 5.08,13.59 5.18,13.59 IC3.3
  Bottom 0.61: U1.3 U1.2 U1.1 25.27,54.48 25.4,54.61 | v34.29,48.26 30.58,48.26 R7.1 | U1.16 34.11,52.38 v34.16,52.32 | U$3.1 8.51,67.06 9.53,66.04 13.08,66.04 13.34,65.79 15.75,65.79 15.88,65.91 20.95,65.91 21.08,66.04 v24.89,66.04 | v27.18,66.04 28.55,66.04 R8.1 | v42.42,19.43 41.4,19.43 39.5,21.34 39.5,22.86 38.35,24 U$1.P$4 | v45.09,19.56 45.09,25.27 44.96,25.4 v44.96,26.92 44.96,33.91 45.21,34.16 45.21,37.21 44.96,37.47 44.96,39.24 45.85,40.13 v47.5,40.13
  Bottom 0.813: C47.1 11.81,61.59 11.18,60.96 v10.67,60.96 | 28.55,52.07 28.55,53.37 28.07,53.85 28.07,65.05 R8.1 | R7.1 R6.1
  Bottom 1.016: v3.43,13.59 4.19,14.35 5.08,14.35 5.08,13.59 | C52.1 v29.59,21.46 | 25.91,6.22 26.04,6.35 26.04,12.32 v27.3,13.59 | C50.+ 24.51,4.83 25.91,6.22 | 25.91,6.22 25.91,8.13 19.05,8.13 v18.67,8.51
  Bottom 1.27: JP1.1 10.79,4.57 9.14,6.22 X1.2

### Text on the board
Top: Master / Controller | Ver 1.0
Bottom: Designed by / Sunny Lee
tPlace: GND | RROUT | RLOUT | COUT | ROUT | LOUT | SC1 | SD1 | SC0 | SC1 | SD1 | SCL | SD0 | SC0 | SD0 | SDA | RMIX | GND | LMIX
bPlace: A0 | 1 0 | A1 | A2 | 0805 | GND | GND | 5V | 9V | -5V | +5V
